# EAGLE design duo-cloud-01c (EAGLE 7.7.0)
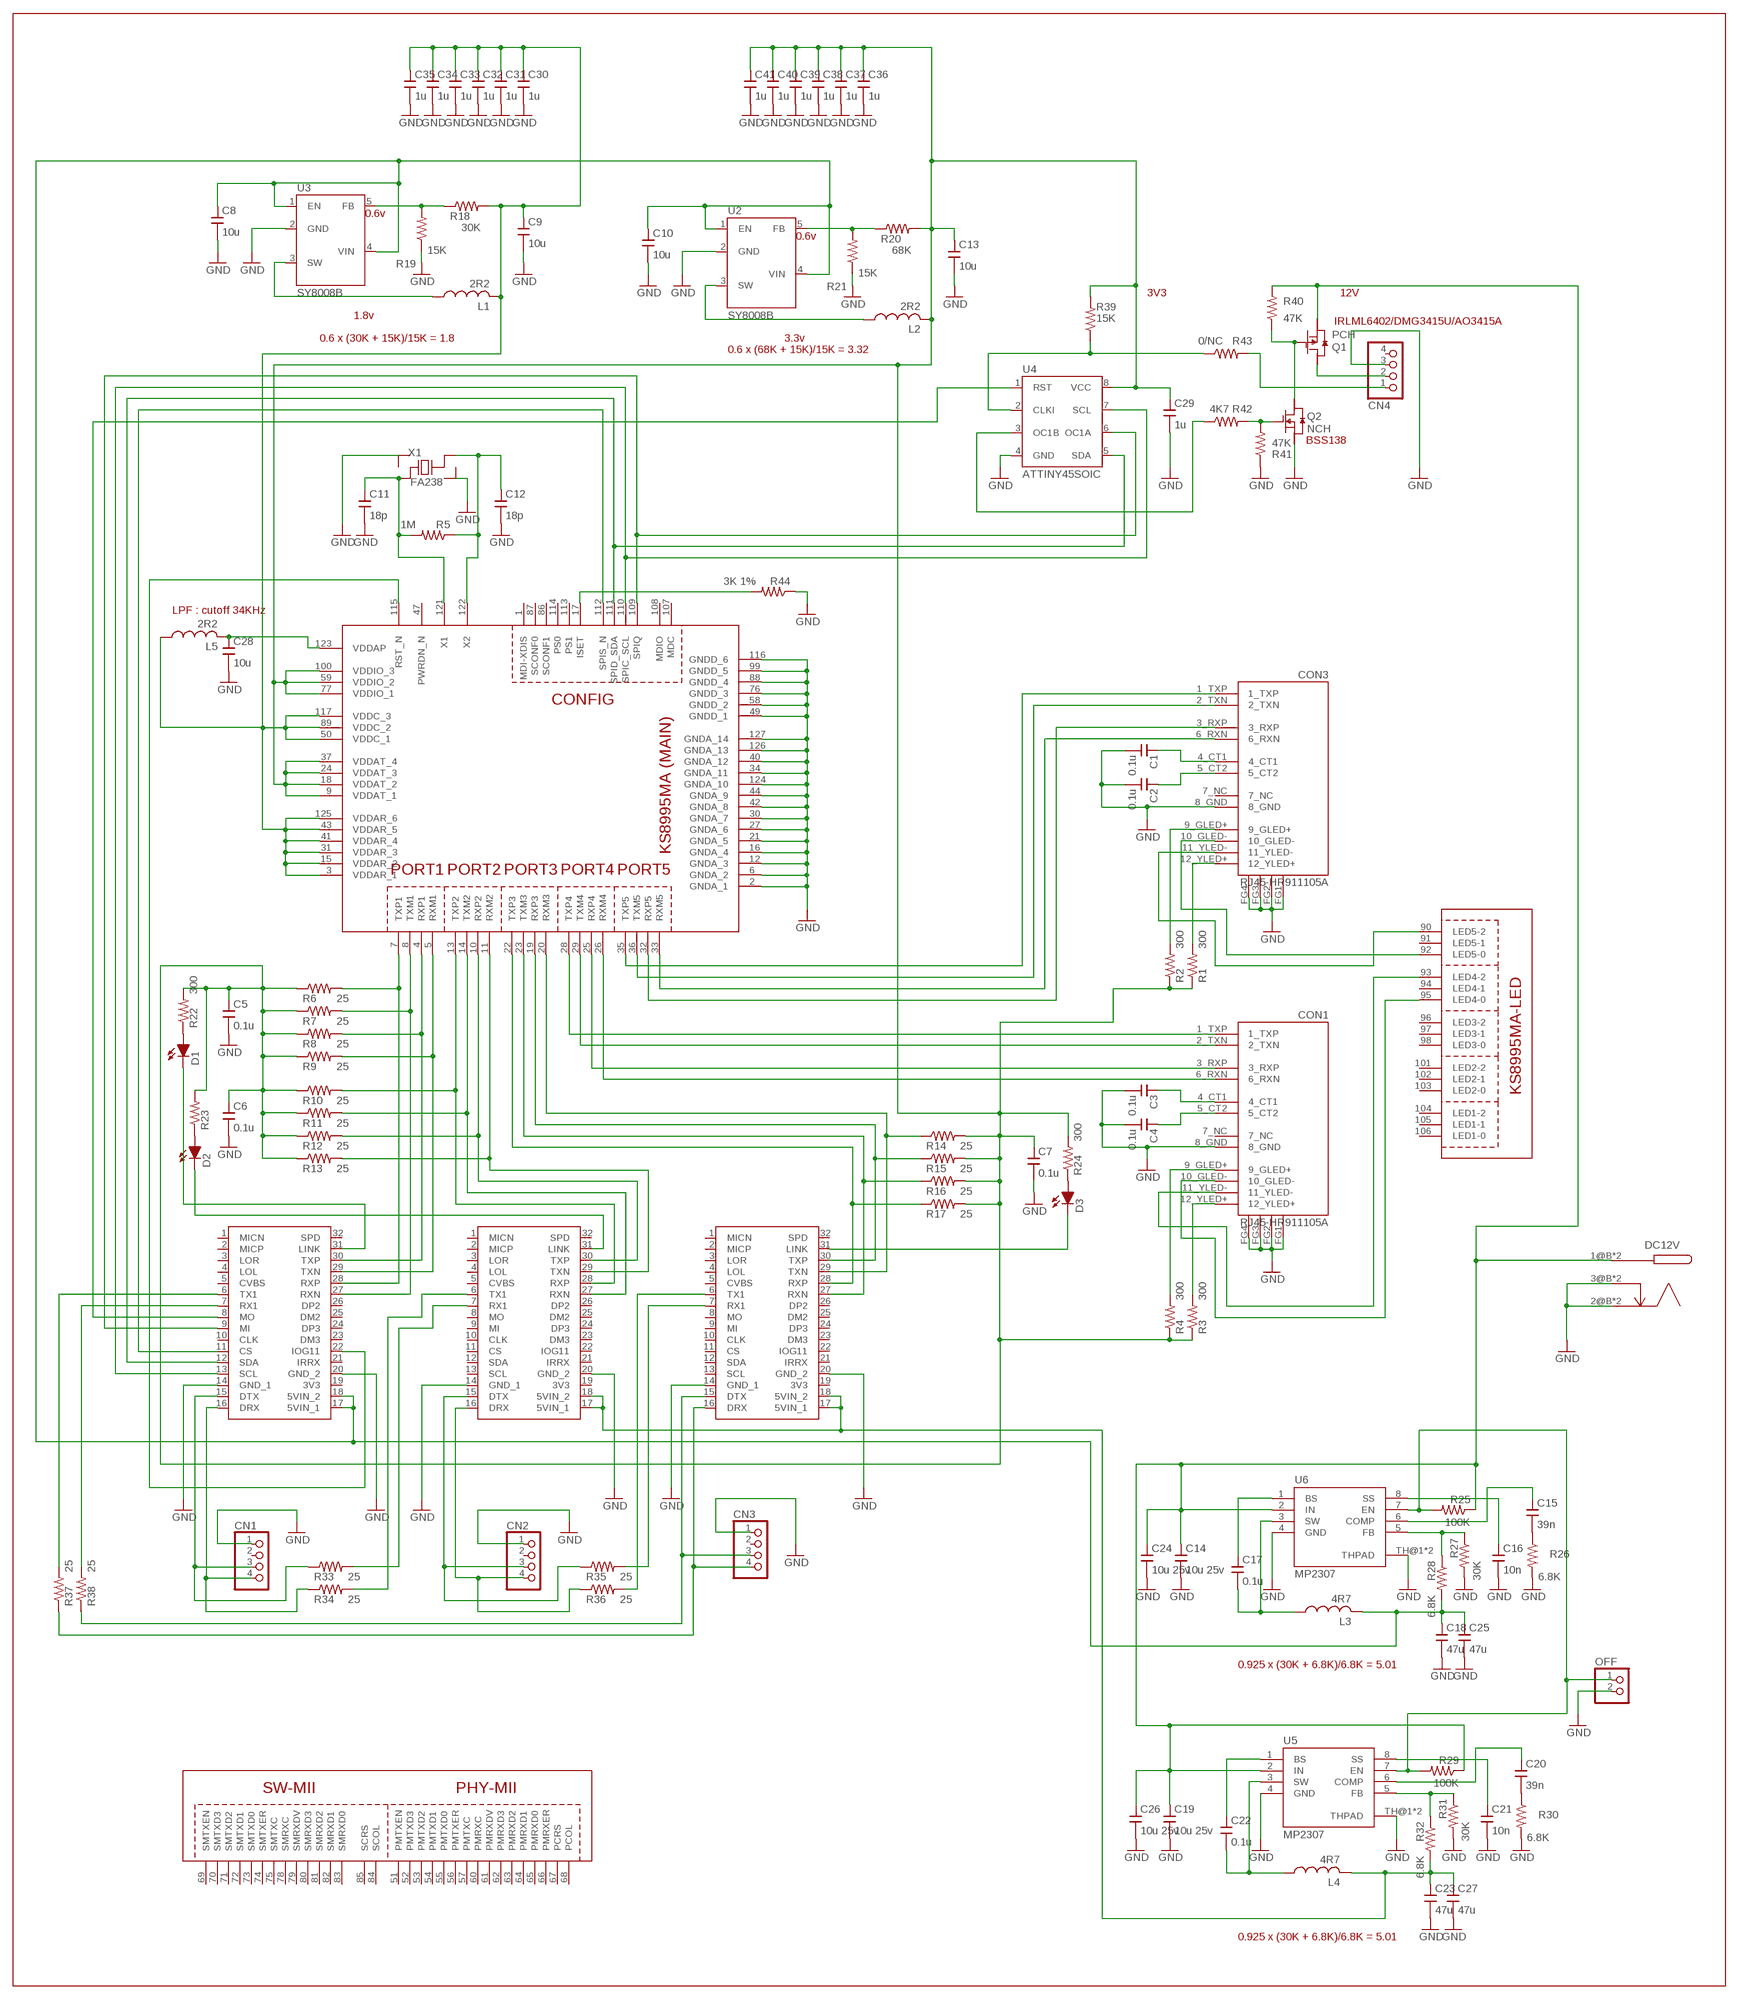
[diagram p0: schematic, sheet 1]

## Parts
C1  0.1u  C/SMDC2012  [C2012]
C2  0.1u  C/SMDC2012  [C2012]
C3  0.1u  C/SMDC2012  [C2012]
C4  0.1u  C/SMDC2012  [C2012]
C5  0.1u  C/SMDC2012  [C2012]
C6  0.1u  C/SMDC2012  [C2012]
C7  0.1u  C/SMDC2012  [C2012]
C8  10u  C/SMDC2012  [C2012]
C9  10u  C/SMDC2012  [C2012]
C10  10u  C/SMDC2012  [C2012]
C11  18p  C/SMDC2012  [C2012]
C12  18p  C/SMDC2012  [C2012]
C13  10u  C/SMDC2012  [C2012]
C14  10u 25v  C/SMDC3216  [C3216]
C15  39n  C/SMDC2012  [C2012]
C16  10n  C/SMDC2012  [C2012]
C17  0.1u  C/SMDC2012  [C2012]
C18  47u  C/SMDC3216  [C3216]
C19  10u 25v  C/SMDC3216  [C3216]
C20  39n  C/SMDC2012  [C2012]
C21  10n  C/SMDC2012  [C2012]
C22  0.1u  C/SMDC2012  [C2012]
C23  47u  C/SMDC3216  [C3216]
C24  10u 25v  C/SMDC3216  [C3216]
C25  47u  C/SMDC3216  [C3216]
C26  10u 25v  C/SMDC3216  [C3216]
C27  47u  C/SMDC3216  [C3216]
C28  10u  C/SMDC2012  [C2012]
C29  1u  C/SMDC2012  [C2012]
C30  1u  C/SMDC2012  [C2012]
C31  1u  C/SMDC2012  [C2012]
C32  1u  C/SMDC2012  [C2012]
C33  1u  C/SMDC2012  [C2012]
C34  1u  C/SMDC2012  [C2012]
C35  1u  C/SMDC2012  [C2012]
C36  1u  C/SMDC2012  [C2012]
C37  1u  C/SMDC2012  [C2012]
C38  1u  C/SMDC2012  [C2012]
C39  1u  C/SMDC2012  [C2012]
C40  1u  C/SMDC2012  [C2012]
C41  1u  C/SMDC2012  [C2012]
CN1  CONN4N  [PINHDR1X4]
CN2  CONN4N  [PINHDR1X4]
CN3  CONN4N  [PINHDR1X4]
CN4  CONN4N  [PINHDR1X4]
CON1  RJ45-HR911105A  [RJ45-HR911105A]
CON3  RJ45-HR911105A  [RJ45-HR911105A]
D1  LED/SMDSMD  [SOD123]
D2  LED/SMDSMD  [SOD123]
D3  LED/SMDSMD  [SOD123]
DC12V  DC-JACK7  [DC-JACK7]
L1  2R2  L/SMDCD54  [CD54]
L2  2R2  L/SMDCD54  [CD54]
L3  4R7  L/SMD  [L10040]
L4  4R7  L/SMD  [L10040]
L5  2R2  L/SMDCD32  [CD32]
M1  NANOPI-DUO  [NANOPI-DUO]
M2  NANOPI-DUO  [NANOPI-DUO]
M3  NANOPI-DUO  [NANOPI-DUO]
OFF  PINHDR2  [PINHDR2]
Q1  PCH  [SOT23]
Q2  NCH  [SOT23]
R1  300  R/SMDR2012  [R2012]
R2  300  R/SMDR2012  [R2012]
R3  300  R/SMDR2012  [R2012]
R4  300  R/SMDR2012  [R2012]
R5  1M  R/SMDR2012  [R2012]
R6  25  R/SMDR2012  [R2012]
R7  25  R/SMDR2012  [R2012]
R8  25  R/SMDR2012  [R2012]
R9  25  R/SMDR2012  [R2012]
R10  25  R/SMDR2012  [R2012]
R11  25  R/SMDR2012  [R2012]
R12  25  R/SMDR2012  [R2012]
R13  25  R/SMDR2012  [R2012]
R14  25  R/SMDR2012  [R2012]
R15  25  R/SMDR2012  [R2012]
R16  25  R/SMDR2012  [R2012]
R17  25  R/SMDR2012  [R2012]
R18  30K  R/SMDR2012  [R2012]
R19  15K  R/SMDR2012  [R2012]
R20  68K  R/SMDR2012  [R2012]
R21  15K  R/SMDR2012  [R2012]
R22  300  R/SMDR2012  [R2012]
R23  300  R/SMDR2012  [R2012]
R24  300  R/SMDR2012  [R2012]
R25  100K  R/SMDR2012  [R2012]
R26  6.8K  R/SMDR2012  [R2012]
R27  30K  R/SMDR2012  [R2012]
R28  6.8K  R/SMDR2012  [R2012]
R29  100K  R/SMDR2012  [R2012]
R30  6.8K  R/SMDR2012  [R2012]
R31  30K  R/SMDR2012  [R2012]
R32  6.8K  R/SMDR2012  [R2012]
R33  25  R/SMDR2012  [R2012]
R34  25  R/SMDR2012  [R2012]
R35  25  R/SMDR2012  [R2012]
R36  25  R/SMDR2012  [R2012]
R37  25  R/SMDR2012  [R2012]
R38  25  R/SMDR2012  [R2012]
R39  15K  R/SMDR2012  [R2012]
R40  47K  R/SMDR2012  [R2012]
R41  47K  R/SMDR2012  [R2012]
R42  4K7  R/SMDR2012  [R2012]
R43  0/NC  R/SMDR2012  [R2012]
R44  3K 1%  R/SMDR2012  [R2012]
U1  KS8995MA+MII  [QFP128]
U2  SY8008B  [SOT235]
U3  SY8008B  [SOT235]
U4  ATTINY45SOIC  [SOIC8]
U5  MP2307  [SOP8PAD]
U6  MP2307  [SOP8PAD]
X1  FA238  [FA238]

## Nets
5VM: C8.1 C10.1 C18.1 C25.1 L3.2 L3.2B M1.17(5VIN_1) M1.18(5VIN_2) R28.2 U2.1(EN) U2.4(VIN) U3.1(EN) U3.4(VIN)
5VS: C23.1 C27.1 L4.2 L4.2B M2.17(5VIN_1) M2.18(5VIN_2) M3.17(5VIN_1) M3.18(5VIN_2) R32.2
CS: M1.11(CS) U1.112(SPIS_N)
GND: C1.2 C2.2 C3.2 C4.2 C5.2 C6.2 C7.2 C8.2 C9.2 C10.2 C11.2 C12.2 C13.2 C14.2 C16.2 C18.2 C19.2 C21.2 C23.2 C24.2 C25.2 C26.2 C27.2 C28.2 C29.2 C30.2 C31.2 C32.2 C33.2 C34.2 C35.2 C36.2 C37.2 C38.2 C39.2 C40.2 C41.2 CN1.1 CN2.1 CN3.1 CN4.3 CON1.8_GND CON1.FG1(GND) CON1.FG2(GND) CON1.FG3(GND) CON1.FG4(GND) CON3.8_GND CON3.FG1(GND) CON3.FG2(GND) CON3.FG3(GND) CON3.FG4(GND) DC12V.2@B(GND) DC12V.2@T(GND) DC12V.3@B(SENSE) DC12V.3@T(SENSE) M1.14(GND_1) M1.20(GND_2) M2.14(GND_1) M2.20(GND_2) M3.14(GND_1) M3.20(GND_2) OFF.2 Q2.2(S) R19.1 R21.1 R26.2 R27.2 R30.2 R31.2 R41.1 R44.1 U1.2(GNDA_1) U1.6(GNDA_2) U1.12(GNDA_3) U1.16(GNDA_4) U1.21(GNDA_5) U1.27(GNDA_6) U1.30(GNDA_7) U1.34(GNDA_11) U1.40(GNDA_12) U1.42(GNDA_8) U1.44(GNDA_9) U1.49(GNDD_1) U1.58(GNDD_2) U1.76(GNDD_3) U1.88(GNDD_4) U1.99(GNDD_5) U1.116(GNDD_6) U1.124(GNDA_10) U1.126(GNDA_13) U1.127(GNDA_14) U2.2(GND) U3.2(GND) U4.4(GND) U5.4(GND) U5.TH@1(THPAD) U5.TH@2(THPAD) U6.4(GND) U6.TH@1(THPAD) U6.TH@2(THPAD) X1.2 X1.4
HUB_1V8: C9.1 C30.1 C31.1 C32.1 C33.1 C34.1 C35.1 L1.2B L1.P$2 L5.1 L5.1B R18.2 U1.3(VDDAR_1) U1.15(VDDAR_2) U1.31(VDDAR_3) U1.41(VDDAR_4) U1.43(VDDAR_5) U1.50(VDDC_1) U1.89(VDDC_2) U1.117(VDDC_3) U1.125(VDDAR_6)
HUB_3V3: C5.1 C6.1 C7.1 C13.1 C29.1 C36.1 C37.1 C38.1 C39.1 C40.1 C41.1 L2.2B L2.P$2 R1.1 R2.1 R3.1 R4.1 R6.1 R7.1 R8.1 R9.1 R10.1 R11.1 R12.1 R13.1 R14.2 R15.2 R16.2 R17.2 R20.2 R22.2 R23.2 R24.2 R39.2 U1.9(VDDAT_1) U1.18(VDDAT_2) U1.24(VDDAT_3) U1.37(VDDAT_4) U1.59(VDDIO_2) U1.77(VDDIO_1) U1.100(VDDIO_3) U4.8(VCC)
HUBRST_N: M1.22(IOG11) U1.115(RST_N)
L1SW: L1.1B L1.P$1 U3.3(SW)
L2SW: L2.1B L2.P$1 U2.3(SW)
MI: M1.9(MI) U1.109(SPIQ) U4.6(OC1A)
N$1: CN4.1 R43.2
N$2: M1.28(RXP) R6.2 U1.7(TXP1)
N$3: M1.27(RXN) R7.2 U1.8(TXM1)
N$4: M1.30(TXP) R8.2 U1.4(RXP1)
N$5: M1.29(TXN) R9.2 U1.5(RXM1)
N$6: M2.28(RXP) R10.2 U1.13(TXP2)
N$7: M2.27(RXN) R11.2 U1.14(TXM2)
N$8: CON3.10_GLED- U1.92(LED5-0)
N$9: M2.30(TXP) R12.2 U1.10(RXP2)
N$10: M2.29(TXN) R13.2 U1.11(RXM2)
N$11: M3.28(RXP) R17.1 U1.22(TXP3)
N$12: M3.27(RXN) R16.1 U1.23(TXM3)
N$13: M3.30(TXP) R15.1 U1.19(RXP3)
N$14: M3.29(TXN) R14.1 U1.20(RXM3)
N$15: CON3.6_RXN U1.33(RXM5)
N$16: CON3.3_RXP U1.32(RXP5)
N$17: CON3.2_TXN U1.36(TXM5)
N$18: CON3.1_TXP U1.35(TXP5)
N$19: C4.1 CON1.5_CT2
N$20: C3.1 CON1.4_CT1
N$21: CON1.9_GLED+ R4.2
N$22: CON1.12_YLED+ R3.2
N$23: OFF.1 R25.2 R29.2 U5.7(EN) U6.7(EN)
N$24: CON1.6_RXN U1.26(RXM4)
N$25: CON1.3_RXP U1.25(RXP4)
N$26: CON1.2_TXN U1.29(TXM4)
N$27: CON1.1_TXP U1.28(TXP4)
N$28: D1.1(A) R22.1
N$29: D2.1(A) R23.1
N$30: D3.1(A) R24.1
N$31: D3.2(C) M3.31(LINK)
N$32: D2.2(C) M2.31(LINK)
N$33: C1.1 CON3.4_CT1
N$34: C2.1 CON3.5_CT2
N$35: D1.2(C) M1.31(LINK)
N$36: CON3.9_GLED+ R2.2
N$37: CON3.12_YLED+ R1.2
N$38: C17.2 L3.1 L3.1B U6.3(SW)
N$39: C17.1 U6.1(BS)
N$40: CON3.11_YLED- U1.90(LED5-2)
N$41: CON1.10_GLED- U1.95(LED4-0)
N$42: CON1.11_YLED- U1.93(LED4-2)
N$43: C28.1 L5.2 L5.2B U1.123(VDDAP)
N$44: CN1.4 M1.16(DRX) R34.1
N$45: C22.2 L4.1 L4.1B U5.3(SW)
N$46: CN1.3 M1.15(DTX) R33.1
N$47: CN3.4 M3.16(DRX) R37.1
N$48: R18.1 R19.2 U3.5(FB)
N$49: C16.1 U6.8(SS)
N$50: C15.2 R26.1
N$51: R20.1 R21.2 U2.5(FB)
N$52: C15.1 U6.6(COMP)
N$53: C11.1 R5.2 U1.121(X1) X1.1
N$54: C12.1 R5.1 U1.122(X2) X1.3
N$55: R27.1 R28.1 U6.5(FB)
N$56: CN2.4 M2.16(DRX) R36.1
N$57: R39.1 R43.1 U4.2(CLKI)
N$58: C21.1 U5.8(SS)
N$59: C20.2 R30.1
N$60: C20.1 U5.6(COMP)
N$61: R31.1 R32.1 U5.5(FB)
N$62: CN2.3 M2.15(DTX) R35.1
N$63: C22.1 U5.1(BS)
N$64: CN3.3 M3.15(DTX) R38.1
N$65: M1.8(MO) U4.1(RST)
N$66: M2.6(TX1) R34.2
N$67: M2.7(RX1) R33.2
N$68: M3.6(TX1) R36.2
N$69: M3.7(RX1) R35.2
N$70: M1.6(TX1) R37.2
N$71: M1.7(RX1) R38.2
N$72: R44.2 U1.17(ISET)
N$73: CN4.2 Q1.3(D)
N$76: Q2.1(G) R41.2 R42.2
N$77: Q1.1(G) Q2.3(D) R40.1
N$78: R42.1 U4.3(OC1B)
SCL: M1.13(SCL) U1.110(SPIC_SCL) U4.7(SCL)
SDA: M1.12(SDA) U1.111(SPID_SDA) U4.5(SDA)
VIN: C14.1 C19.1 C24.1 C26.1 DC12V.1@B(VIN) DC12V.1@T(VIN) Q1.2(S) R25.1 R29.1 R40.2 U5.2(IN) U6.2(IN)
Unconnected: CN1.2 CN2.2 CN3.2 CN4.4 CON1.7_NC CON3.7_NC M1.1(MICN) M1.2(MICP) M1.3(LOR) M1.4(LOL) M1.5(CVBS) M1.10(CLK) M1.19(3V3) M1.21(IRRX) M1.23(DM3) M1.24(DP3) M1.25(DM2) M1.26(DP2) M1.32(SPD) M2.1(MICN) M2.2(MICP) M2.3(LOR) M2.4(LOL) M2.5(CVBS) M2.8(MO) M2.9(MI) M2.10(CLK) M2.11(CS) M2.12(SDA) M2.13(SCL) M2.19(3V3) M2.21(IRRX) M2.22(IOG11) M2.23(DM3) M2.24(DP3) M2.25(DM2) M2.26(DP2) M2.32(SPD) M3.1(MICN) M3.2(MICP) M3.3(LOR) M3.4(LOL) M3.5(CVBS) M3.8(MO) M3.9(MI) M3.10(CLK) M3.11(CS) M3.12(SDA) M3.13(SCL) M3.19(3V3) M3.21(IRRX) M3.22(IOG11) M3.23(DM3) M3.24(DP3) M3.25(DM2) M3.26(DP2) M3.32(SPD) U1.1(MDI-XDIS) U1.47(PWRDN_N) U1.51(PMTXEN) U1.52(PMTXD3) U1.53(PMTXD2) U1.54(PMTXD1) U1.55(PMTXD0) U1.56(PMTXER) U1.57(PMTXC) U1.60(PMRXC) U1.61(PMRXDV) U1.62(PMRXD3) U1.63(PMRXD2) U1.64(PMRXD1) U1.65(PMRXD0) U1.66(PMRXER) U1.67(PCRS) U1.68(PCOL) U1.69(SMTXEN) U1.70(SMTXD3) U1.71(SMTXD2) U1.72(SMTXD1) U1.73(SMTXD0) U1.74(SMTXER) U1.75(SMTXC) U1.78(SMRXC) U1.79(SMRXDV) U1.80(SMRXD3) U1.81(SMRXD2) U1.82(SMRXD1) U1.83(SMRXD0) U1.84(SCOL) U1.85(SCRS) U1.86(SCONF1) U1.87(SCONF0) U1.91(LED5-1) U1.94(LED4-1) U1.96(LED3-2) U1.97(LED3-1) U1.98(LED3-0) U1.101(LED2-2) U1.102(LED2-1) U1.103(LED2-0) U1.104(LED1-2) U1.105(LED1-1) U1.106(LED1-0) U1.107(MDC) U1.108(MDIO) U1.113(PS1) U1.114(PS0)

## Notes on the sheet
- 0.6v
- 0.6v
- 3V3 | 12V
- 1.8v
- IRLML6402/DMG3415U/AO3415A
- 0.6 x (30K + 15K)/15K = 1.8 | 3.3v
- 0.6 x (68K + 15K)/15K = 3.32
- BSS138
- LPF : cutoff 34KHz
- 0.925 x (30K + 6.8K)/6.8K = 5.01
- 0.925 x (30K + 6.8K)/6.8K = 5.01

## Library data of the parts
C1-C41 = SRT162-020:C/SMD
CN1-CN4 = SRT162-020:CONN4: connector 4
CON1 CON3 = SRT162-020:RJ45-HR911105A
D1-D3 = SRT162-020:LED/SMD
DC12V = SRT162-020:DC-JACK
L1-L5 = SRT162-020:L/SMD: VLF4012AT
M1-M3 = SRT162-020:NANOPI-DUO
OFF = SRT162-020:PINHDR2
Q1 = SRT162-020:PCH
Q2 = SRT162-020:NCH
R1-R44 = SRT162-020:R/SMD
U1 = SRT162-020:KS8995MA+MII
U2 U3 = SRT162-020:SY8008B
U4 = SRT162-020:ATTINY45
U5 U6 = SRT162-020:MP2307
X1 = SRT162-020:FA238

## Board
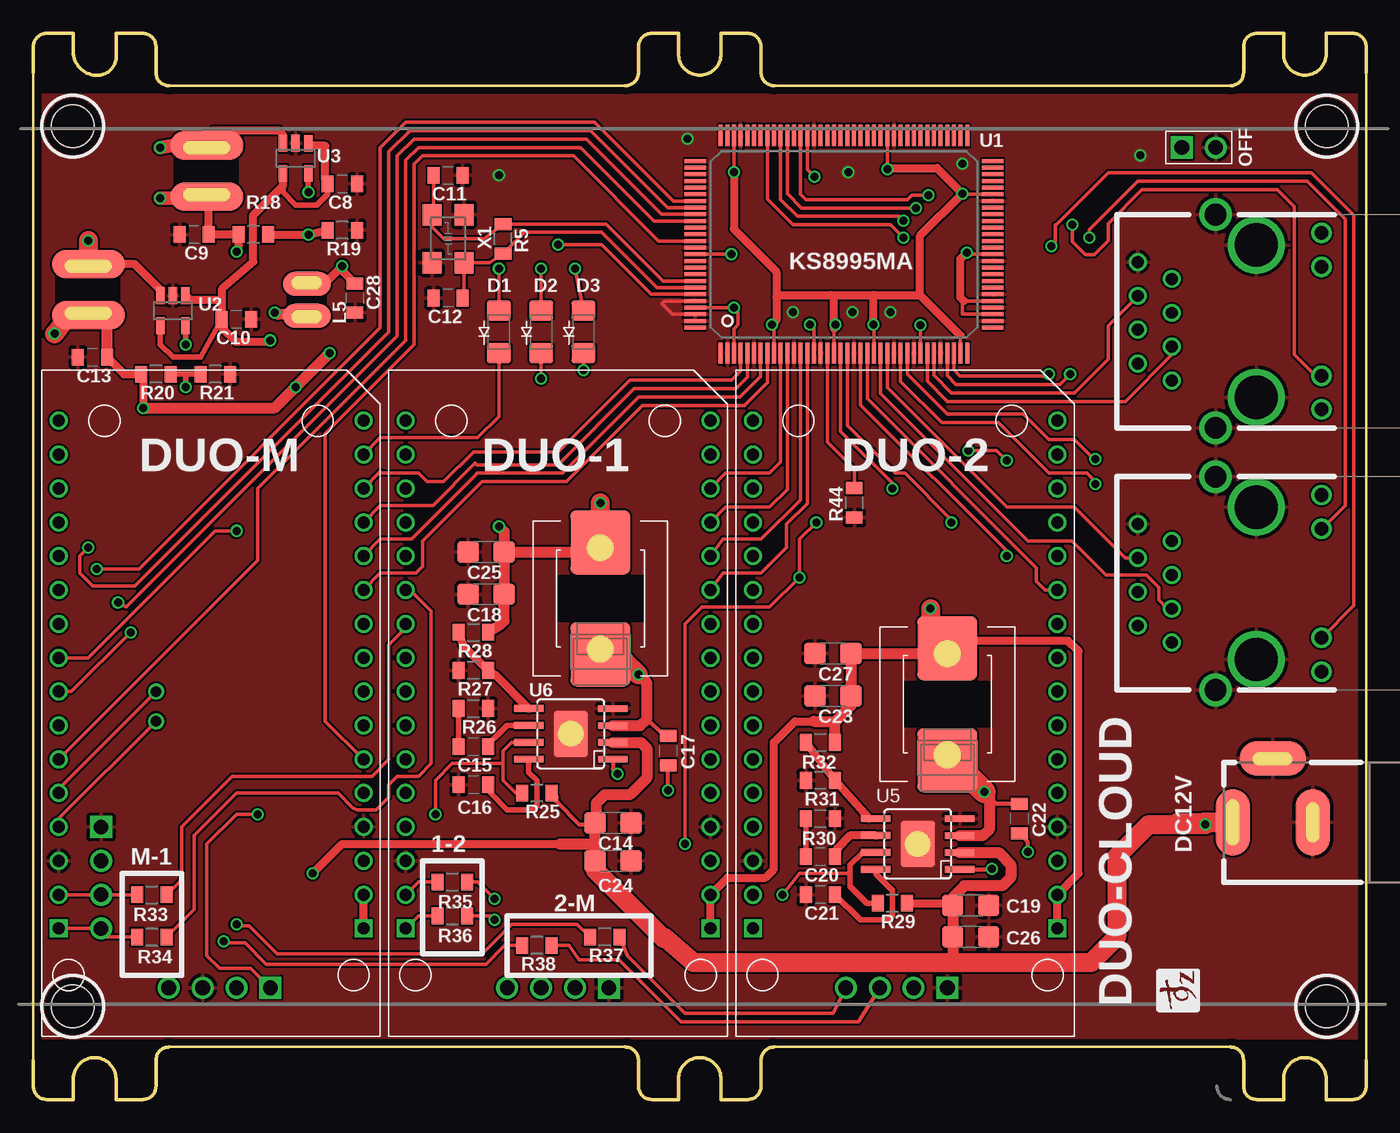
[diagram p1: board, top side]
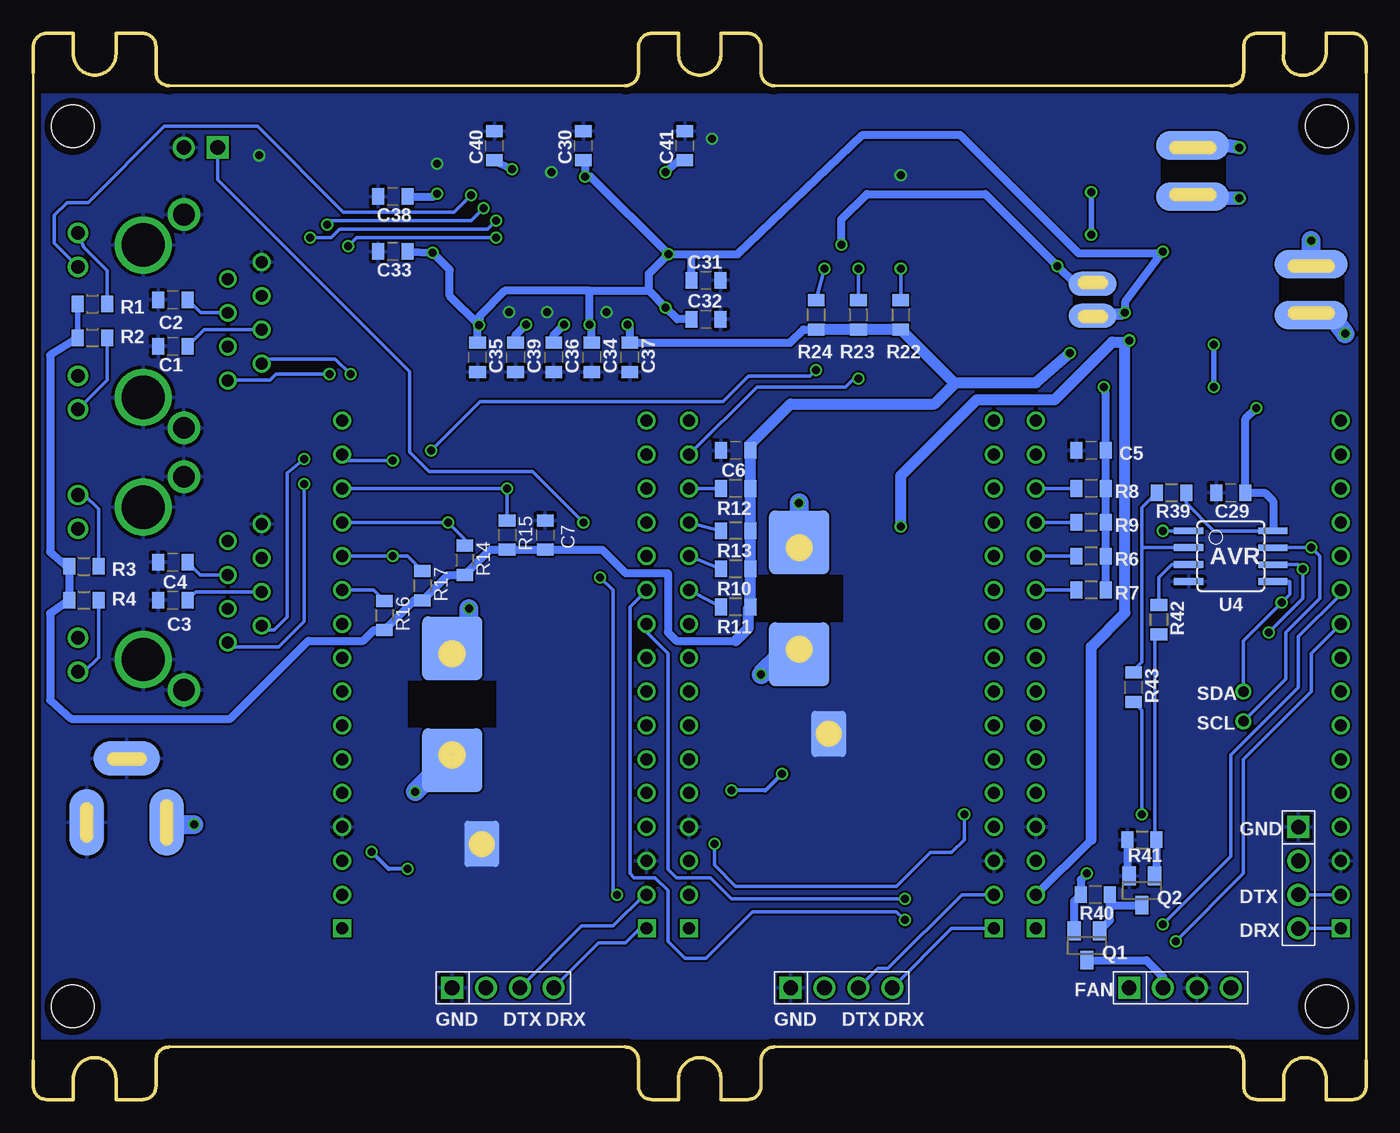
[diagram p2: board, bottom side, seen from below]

Size 100 x 80 mm. Coordinates in mm from the lower left corner, seen from the top.
Outline: 75 segments
Copper layers (1*16): Top 0.035mm / dielectric 1.6mm / Bottom 0.035mm
Design rules "Elecrow_2-layer_PCB_eagle_rule": minimum track width 6mil, minimum drill 12mil, track to track 6mil, track to pad 6mil, pad to pad 6mil, via to via 8mil, smd to smd 0mil, copper to edge 20mil, drill to drill 10mil, minimum pad ring 6mil, minimum via ring 6mil, stop-mask expansion 0mil, vias tented up to drill 100mil, thermal gap 10mil
Holes 3.2 mm at 2.97,73.02 97.05,73.02 2.97,6.98 97.05,6.98
tRestrict: area -4,-1 to 103,4.5; area -3,75.5 to 104,81
bRestrict: area -4,-1 to 103,4.5; area -3,75.5 to 104,81

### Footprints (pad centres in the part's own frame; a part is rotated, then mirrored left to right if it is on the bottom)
C2012 = smd 0.9 x 1.25: 1 -1.1,0; 2 1.1,0
C3216 = smd 1.6 x 1.6: 1 -1.35,0; 2 1.35,0
PINHDR1X4 = drill 1.1 square: 1 -3.81,0 | drill 1.1: 2 -1.27,0; 3 1.27,0; 4 3.81,0
RJ45-HR911105A = drill 0.89 pad 1.144: 1_TXP 4.45,-6.35; 2_TXN 3.18,-8.89; 3_RXP 1.91,-6.35; 4_CT1 0.64,-8.89; 5_CT2 -0.63,-6.35; 6_RXN -1.9,-8.89; 7_NC -3.17,-6.35; 8_GND -4.44,-8.89 | drill 1.02 pad 1.528: 9_GLED+ 6.625,4.9; 10_GLED- 4.085,4.9; 11_YLED- -4.085,4.9; 12_YLED+ -6.625,4.9 | drill 1.63: FG1 8,-3.05; FG2 -8,-3.05 | drill 3.25 pad 3.75: FG3 5.715,0; FG4 -5.715,0
SOD123 = smd 1.5 x 1.8: 1 -1.6,0; 2 1.6,0
DC-JACK7 = smd 2.6 x 5 bottom: 1@B 4,0; 2@B -2,0 | smd 2.6 x 5: 1@T 4,0; 2@T -2,0 | smd 5 x 2.6 bottom: 3@B 1,-4.8 | smd 5 x 2.6: 3@T 1,-4.8
CD54 = smd 5.5 x 2.15 bottom: 1B 0,1.925; 2B 0,-1.925 | smd 5.5 x 2.15: P$1 0,1.925; P$2 0,-1.925
L10040 = smd 4.5 x 4.8: 1 0,4.2; 2 0,-4.2 | smd 4.5 x 4.8 bottom: 1B 0,4.2; 2B 0,-4.2
CD32 = smd 1.8 x 3.6: 1 -1.2,0; 2 1.2,0 | smd 1.8 x 3.6 bottom: 1B -1.2,0; 2B 1.2,0
NANOPI-DUO = drill 0.9: 1 -10.16,10.16; 2 -10.16,7.62; 3 -10.16,5.08; 4 -10.16,2.54; 5 -10.16,0; 6 -10.16,-2.54; 7 -10.16,-5.08; 8 -10.16,-7.62; 9 -10.16,-10.16; 10 -10.16,-12.7; 11 -10.16,-15.24; 12 -10.16,-17.78; 13 -10.16,-20.32; 14 -10.16,-22.86; 15 -10.16,-25.4; 18 12.7,-25.4; 19 12.7,-22.86; 20 12.7,-20.32; 21 12.7,-17.78; 22 12.7,-15.24; 23 12.7,-12.7; 24 12.7,-10.16; 25 12.7,-7.62; 26 12.7,-5.08; 27 12.7,-2.54; 28 12.7,0; 29 12.7,2.54; 30 12.7,5.08; 31 12.7,7.62; 32 12.7,10.16 | drill 0.9 square: 16 -10.16,-27.94; 17 12.7,-27.94
PINHDR2 = drill 1.1 square: 1 -1.27,0 | drill 1.1: 2 1.27,0
SOT23 = smd 1 x 1.4: 1 -0.95,-1.1; 2 0.95,-1.1; 3 0,1.1
R2012 = smd 0.9 x 1.25: 1 -1.1,0; 2 1.1,0
QFP128 = smd 0.3 x 1.6: 1 -9.25,-8.16; 2 -8.75,-8.16; 3 -8.25,-8.16; 4 -7.75,-8.16; 5 -7.25,-8.16; 6 -6.75,-8.16; 7 -6.25,-8.16; 8 -5.75,-8.16; 9 -5.25,-8.16; 10 -4.75,-8.16; 11 -4.25,-8.16; 12 -3.75,-8.16; 13 -3.25,-8.16; 14 -2.75,-8.16; 15 -2.25,-8.16; 16 -1.75,-8.16; 17 -1.25,-8.16; 18 -0.75,-8.16; 19 -0.25,-8.16; 20 0.25,-8.16; 21 0.75,-8.16; 22 1.25,-8.16; 23 1.75,-8.16; 24 2.25,-8.16; 25 2.75,-8.16; 26 3.25,-8.16; 27 3.75,-8.16; 28 4.25,-8.16; 29 4.75,-8.16; 30 5.25,-8.16; 31 5.75,-8.16; 32 6.25,-8.16; 33 6.75,-8.16; 34 7.25,-8.16; 35 7.75,-8.16; 36 8.25,-8.16; 37 8.75,-8.16; 38 9.25,-8.16; 65 9.25,8.16; 66 8.75,8.16; 67 8.25,8.16; 68 7.75,8.16; 69 7.25,8.16; 70 6.75,8.16; 71 6.25,8.16; 72 5.75,8.16; 73 5.25,8.16; 74 4.75,8.16; 75 4.25,8.16; 76 3.75,8.16; 77 3.25,8.16; 78 2.75,8.16; 79 2.25,8.16; 80 1.75,8.16; 81 1.25,8.16; 82 0.75,8.16; 83 0.25,8.16; 84 -0.25,8.16; 85 -0.75,8.16; 86 -1.25,8.16; 87 -1.75,8.16; 88 -2.25,8.16; 89 -2.75,8.16; 90 -3.25,8.16; 91 -3.75,8.16; 92 -4.25,8.16; 93 -4.75,8.16; 94 -5.25,8.16; 95 -5.75,8.16; 96 -6.25,8.16; 97 -6.75,8.16; 98 -7.25,8.16; 99 -7.75,8.16; 100 -8.25,8.16; 101 -8.75,8.16; 102 -9.25,8.16 | smd 1.6 x 0.3: 39 11.16,-6.25; 40 11.16,-5.75; 41 11.16,-5.25; 42 11.16,-4.75; 43 11.16,-4.25; 44 11.16,-3.75; 45 11.16,-3.25; 46 11.16,-2.75; 47 11.16,-2.25; 48 11.16,-1.75; 49 11.16,-1.25; 50 11.16,-0.75; 51 11.16,-0.25; 52 11.16,0.25; 53 11.16,0.75; 54 11.16,1.25; 55 11.16,1.75; 56 11.16,2.25; 57 11.16,2.75; 58 11.16,3.25; 59 11.16,3.75; 60 11.16,4.25; 61 11.16,4.75; 62 11.16,5.25; 63 11.16,5.75; 64 11.16,6.25; 103 -11.16,6.25; 104 -11.16,5.75; 105 -11.16,5.25; 106 -11.16,4.75; 107 -11.16,4.25; 108 -11.16,3.75; 109 -11.16,3.25; 110 -11.16,2.75; 111 -11.16,2.25; 112 -11.16,1.75; 113 -11.16,1.25; 114 -11.16,0.75; 115 -11.16,0.25; 116 -11.16,-0.25; 117 -11.16,-0.75; 118 -11.16,-1.25; 119 -11.16,-1.75; 120 -11.16,-2.25; 121 -11.16,-2.75; 122 -11.16,-3.25; 123 -11.16,-3.75; 124 -11.16,-4.25; 125 -11.16,-4.75; 126 -11.16,-5.25; 127 -11.16,-5.75; 128 -11.16,-6.25
SOT235 = smd 0.635 x 1.27: 1 -0.95,-1.125; 2 0.013,-1.135; 3 0.95,-1.125; 4 0.95,1.125; 5 -0.95,1.125
SOIC8 = smd 0.5 x 2.2: 1 -1.905,-3.154; 2 -0.645,-3.154; 3 0.625,-3.154; 4 1.895,-3.154; 5 1.905,3.154; 6 0.635,3.154; 7 -0.635,3.154; 8 -1.905,3.154
SOP8PAD = smd 0.5 x 2.2: 1 -1.905,-3.154; 2 -0.645,-3.154; 3 0.625,-3.154; 4 1.895,-3.154; 5 1.905,3.154; 6 0.635,3.154; 7 -0.635,3.154; 8 -1.905,3.154 | smd 3.454 x 2.565: TH@1 0,0 | smd 3.454 x 2.565 bottom: TH@2 0,0
FA238 = smd 1.6 x 1.4: 1 -1.8,-1.2; 2 1.8,-1.2; 3 1.8,1.2; 4 -1.8,1.2

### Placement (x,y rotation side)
C1  89.53,56.52 180 bottom
C2  89.53,60.01 180 bottom
C3  89.53,37.47 180 bottom
C4  89.53,40.32 180 bottom
C5  20.64,48.71 180 bottom
C6  47.31,48.71 180 bottom
C7  61.59,42.36 90 bottom
C8  23.18,68.71 0 top
C9  12.06,64.9 180 top
C10  15.24,58.55 0 top
C11  31.11,69.34 0 top
C12  31.11,60.14 180 top
C13  4.45,55.69 180 top
C14  43.5,20.77 0 top
C15  33.02,26.48 180 top
C16  33.02,23.62 180 top
C17  47.62,26.16 90 top
C18  33.97,37.91 180 top
C19  70.33,14.58 0 top
C20  59.05,18.23 180 top
C21  59.05,15.37 180 top
C22  73.98,21.09 90 top
C23  60.01,30.29 180 top
C24  43.5,17.91 0 top
C25  33.97,41.09 180 top
C26  70.33,12.2 0 top
C27  60.01,33.47 180 top
C28  24.13,60.14 270 top
C29  10.16,45.53 180 bottom
C30  58.74,71.57 90 bottom
C31  49.53,61.47 0 bottom
C32  49.53,58.55 0 bottom
C33  73.03,63.63 180 bottom
C34  58.1,55.69 270 bottom
C35  66.67,55.69 270 bottom
C36  60.96,55.69 270 bottom
C37  55.24,55.69 270 bottom
C38  73.03,67.76 180 bottom
C39  63.82,55.69 270 bottom
C40  65.41,71.57 90 bottom
C41  51.12,71.57 90 bottom
CN1  5.08,16.64 270 bottom
CN2  39.37,8.38 0 bottom
CN3  64.77,8.38 0 bottom
CN4  13.97,8.38 0 bottom
CON1  91.76,38.73 270 top
CON3  91.76,58.4 270 top
D1  34.92,57.6 270 top
D2  38.1,57.6 270 top
D3  41.27,57.6 270 top
DC12V  93.98,20.8 180 top
L1  13.02,69.66 0 top
L2  4.13,60.77 0 top
L3  42.55,37.59 180 top
L4  68.58,29.66 180 top
L5  20.51,60.01 90 top
M1  12.06,40.77 0 top
M2  38.1,40.77 0 top
M3  64.14,40.77 0 top
OFF  87.44,71.44 0 top
Q1  20.95,11.56 180 bottom
Q2  16.83,15.69 180 bottom
R1  95.57,59.69 0 bottom
R2  95.57,57.15 0 bottom
R3  96.2,40.01 0 bottom
R4  96.2,37.47 0 bottom
R5  35.24,64.58 90 top
R6  20.64,40.77 180 bottom
R7  20.64,38.23 180 bottom
R8  20.64,45.85 180 bottom
R9  20.64,43.31 180 bottom
R10  47.31,39.82 180 bottom
R11  47.31,36.96 180 bottom
R12  47.31,45.85 180 bottom
R13  47.31,42.67 180 bottom
R14  67.63,40.45 270 bottom
R15  64.45,42.36 270 bottom
R16  73.66,36.33 270 bottom
R17  70.8,38.55 270 bottom
R18  16.51,64.9 180 top
R19  23.18,65.22 180 top
R20  9.21,54.42 180 top
R21  13.65,54.42 180 top
R22  34.92,58.87 270 bottom
R23  38.1,58.87 270 bottom
R24  41.27,58.87 270 bottom
R25  37.78,22.99 180 top
R26  33.02,29.34 0 top
R27  33.02,32.2 180 top
R28  33.02,35.05 0 top
R29  64.45,14.73 180 top
R30  59.05,21.09 0 top
R31  59.05,23.94 180 top
R32  59.05,26.8 0 top
R33  8.89,15.37 0 top
R34  8.89,12.2 0 top
R35  31.43,16.32 0 top
R36  31.43,13.78 0 top
R37  42.86,12.2 180 top
R38  37.78,11.56 180 top
R39  14.61,45.53 0 bottom
R40  20.32,15.37 180 bottom
R41  16.83,19.5 0 bottom
R42  15.56,36.01 270 bottom
R43  17.46,30.93 270 bottom
R44  61.59,44.77 90 top
U1  60.82,64.17 0 top
U2  10.48,59.19 180 top
U3  19.68,70.61 180 top
U4  10.16,40.77 270 bottom
U5  66.36,19.18 90 top
U6  40.32,27.43 90 top
X1  31.11,64.58 270 top

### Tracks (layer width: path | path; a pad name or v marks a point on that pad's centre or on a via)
5VM  (via drill 0.6)
  Top 0.254: 35.01,40.45 35.01,40.69
  Top 0.406: 18.73,68.58 18.73,68.07 19.68,67.12 21.27,67.12 22.08,67.93 C8.1 | 20.81,71.57 U3.1 | 22.23,68.71 21.91,69.03 | U2.4 9.53,56.64 10.48,55.69 12.55,55.69 C10.1 | 35.01,40.69 34.92,40.69
  Top 0.61: 21.91,69.03 21.91,71.57 20.81,71.57 | C8.1 22.23,68.71 | L3.2B 42.94,41.41 | M1.17 M1.18 | L3.2B 42.55,41.27 42.55,40.45 | L3.2B 43.25,41.16 | v17.78,56.96 17.63,56.96 17.5,56.83 15.24,56.83 14.14,57.93 C10.1 14.14,60.01 | U3.4 18.73,68.58 16.51,66.36 16.51,62.85 14.14,60.8 14.14,60.01 | U2.1 11.73,60.01 14.14,60.01 | 35.01,40.69 35.01,40.77 C25.1
  Top 0.813: R28.2 35.01,35.62 35.32,35.94 C18.1 C25.1 | v34.92,42.99 35.32,42.59 C25.1 | C25.1 42.36,41.09 42.55,41.27
  Top 1.422: L3.2B v42.55,44.77
  Top 1.676: 41.52,40.77 L3.2B
  Bottom 0.61: M1.18 20.64,19.5
  Bottom 0.813: v34.92,42.99 34.92,46.8 29.21,52.52 23.36,52.52 19.05,56.83 17.91,56.83 v17.78,56.96 18.1,56.65 18.1,36.51 20.64,33.97 20.64,19.5
  Bottom 1.422: v42.55,44.77 L3.2B 42.55,40.64
5VS  (via drill 0.6)
  Top 0.406: C23.1 61.4,29.62
  Top 0.61: L4.2B 68.78,33.34 69.29,33.15 | 76.52,12.51 M3.17 M3.18 78.42,16.96 78.42,33.66 77.63,34.42 69.17,34.42 L4.2B | L4.2B 68.58,32.52 | M2.17 M2.18 52.07,16.64 54.93,16.64 55.56,17.27 55.56,26.8 57.15,28.39 58.57,28.39
  Top 0.813: C23.1 C27.1 68.19,33.47 L4.2B | 58.57,28.39 60.17,28.39 | 60.17,28.39 61.4,29.62 | R32.2 60.16,28.38 60.17,28.39
  Top 1.422: v67.31,36.83 67.31,34.49 L4.2B
  Bottom 1.422: L4.2B 67.31,33.86 v67.31,36.83
CS
  Top 0.254: M1.11 16.83,40.45 16.83,45.85 27.94,56.96 27.94,70.48 28.89,71.44 41.04,71.44 46.56,65.92 U1.112
GND  (via drill 0.6)
  Top 0.254: U1.124 47.36,59.92 47.17,59.73 47.97,58.92 U1.126
  Bottom 0.254: 17.93,17.25 Q2.2
  Bottom 0.61: R41.1 17.93,17.25
  other vias: 83.05,70.84 49.07,72.11 61.14,69.57 69.71,70.2 61.45,59.09 34.92,69.34 57.01,59.09 64.31,59.09
  pour Bottom: -4.45,86.17 -4.45,-2.82 106.05,-2.82 106.05,86.17
  pour Top: -6.03,87.44 -6.43,-2.2 103.11,-2.2 103.5,88.08 -5.71,88.08
HUB_1V8  (via drill 0.6)
  Top 0.254: U1.117 v52.36,63.42 | U1.125 v52.55,59.42 | v52.55,59.42 52.56,59.41 | U1.3 52.57,57.83 52.88,58.14 52.88,59.09 v52.55,59.42 | U1.15 58.57,57.85 v58.28,58.14 | U1.31 v66.57,58.1 | U1.43 69.83,59.92 69.71,59.92 69.71,58.92 U1.41 | U1.50 70.14,63.42 v70.03,63.53 | U1.89 58.07,69.78 v58.6,69.25
  Top 0.406: v15.24,63.63 15.41,64.09 | 13.16,67.61 13.97,67.44 13.31,67.44 L1.2B
  Top 0.61: 15.41,64.09 R18.2 C9.1 13.16,67.61 | 69.83,59.92 69.55,60.2 69.55,63.06 v70.03,63.53 | L5.1B 18.34,58.81 v18.1,59.05 20.26,59.05 L5.1B
  Top 1.016: v9.53,67.63 12.91,67.63 L1.2B
  Top 1.422: L1.2B 12.38,67.42
  Bottom 0.61: 52.55,63.23 v52.36,63.42 | v66.57,58.1 68.76,60.29 68.76,62.27 v70.03,63.53 C33.1 | 58.28,60.68 64.63,60.68 66.53,58.77 66.53,58.14 v66.57,58.1 | 58.28,60.68 v58.28,58.14 58.1,57.96 C34.1 | v52.36,63.42 50.48,63.42 | 50.48,63.42 47.15,63.42 37.78,72.39 30.48,72.39 21.59,63.5 15.37,63.5 v15.24,63.63 18.1,59.82 v18.1,59.05 | v18.1,59.05 20.26,59.05 L5.1B 18.34,58.81 v18.1,59.05 | C35.1 66.67,58 v66.57,58.1 | v52.36,63.42 58.19,69.25 v58.6,69.25 58.6,70.33 C30.1 | 58.28,60.68 53.81,60.68 | 53.81,60.68 v52.55,59.42 51.68,58.55 C32.1 | 53.81,60.68 53.81,61.97 v52.36,63.42 | C31.1 50.63,63.27 50.48,63.42
  Bottom 1.016: v9.53,67.63 13.02,67.63
  Bottom 1.422: 13.02,67.63 L1.2B
HUB_3V3  (via drill 0.6)
  Top 0.254: U1.59 69.77,67.92 v69.71,67.98 | U1.77 v64.07,69.81 64.31,69.89 | U1.100 52.57,69.89 v52.56,69.57 | U1.9 55.57,57.82 v55.42,58.14 | U1.18 60.07,57.82 v60.19,58.14 | U1.24 63.07,57.82 v63.04,58.14 | U1.37 69.57,57.33
  Top 0.406: 5.54,58.72 5.4,58.87 4.15,58.87 L2.2B
  Top 0.61: 59.87,60.36 55.87,60.36 55.74,60.23 | 59.87,60.36 63.04,60.36 | 63.04,60.36 66.53,60.36 | 66.53,60.36 69.57,57.33 | 60.07,57.82 60.07,60.16 59.87,60.36 | v63.04,58.14 63.04,60.36 | 64.31,69.89 67.81,69.89 v69.71,67.98 66.53,64.81 66.53,60.36 | v52.56,69.57 52.56,65.31 55.74,62.13 55.74,60.23 | 55.74,60.23 55.74,58.45 v55.42,58.14 | C13.1 6.82,54.42 R20.2 8.26,54.27 v8.26,51.88
  Top 0.813: C13.1 5.54,58.72 | v22.23,56.01 v19.68,53.47 18.1,51.88 v8.26,51.88
  Top 1.422: L2.2B 2.65,58.85 v1.59,57.47
  Bottom 0.254: 46.35,37.91 46.52,38.06 R11.1 | v64.07,69.81 64.24,69.81 | 6.99,42.7 U4.8 11.43,42.67 13.51,44.75 R39.2
  Bottom 0.406: R1.1 R2.1 | R3.1 97.47,40.01 97.3,39.84
  Bottom 0.61: R7.1 R6.1 R9.1 R8.1 C5.1 19.54,52.98 v19.68,53.47 | 6.99,42.7 6.99,44.9 7.62,45.53 C29.1 9.06,51.08 v8.26,51.88 | 30.95,53.79 30.8,53.79 | C6.1 46.21,49.17 | 46.35,36.96 46.35,37.91 | R2.1 98.74,55.84 98.74,41.09 97.47,40.01 | 97.3,39.84 R4.1 98.74,36.47 98.74,29.98 97.16,28.57 85.22,28.57 79.38,34.42 75.25,34.42 74.44,35.23 R16.2 71.44,37.45 R17.2 68.9,39.35 R14.2 65.72,41.26 R15.2 C7.1 57.32,41.26 55.56,39.5 52.39,39.5 52.39,35.05 51.75,34.42 47.31,34.42 | 46.35,36.81 R11.1 | 40.96,57.77 R24.2 41.29,57.78 42.23,57.78 43.22,56.79 C37.1 55.24,57.96 v55.42,58.14 | C39.1 63.82,57.36 v63.04,58.14 | C36.1 60.96,57.36 v60.19,58.14 | C38.1 69.93,67.76 v69.71,67.98 | C41.1 51.49,70.52 v52.56,69.57 | C40.1 65.38,70.44 v64.07,69.81
  Bottom 0.813: 40.96,57.77 R23.2 R22.2 30.95,53.79 | R11.1 R10.1 R13.1 R12.1 C6.1 | v22.23,56.01 24.77,53.79 30.8,53.79 32.38,52.2 43.18,52.2 46.21,49.17 | 47.31,34.42 46.35,35.37 46.35,36.81
  Bottom 1.422: v1.59,57.47 2.65,58.85 L2.2B
HUBRST_N
  Top 0.254: M1.22 21.91,28.39 21.91,49.98 28.57,56.65 28.57,70.17 29.21,70.8 40.53,70.8 46.92,64.42 U1.115
L1SW  (via drill 0.6)
  Top 0.406: 18.73,72.2 | 13.04,72.2 L1.1B
  Top 0.61: U3.3 18.73,72.2 18.73,72.39 18.41,72.71 13.5,72.71 L1.1B
  Top 1.016: v9.53,71.44 13.02,72.07
  Top 1.422: 13.02,72.07 L1.1B
  Bottom 1.016: v9.53,71.44 12.87,72.07 L1.1B
L2SW  (via drill 0.6)
  Top 0.406: 4.15,62.68 L2.1B
  Top 0.61: U2.3 9.53,60.77 7.62,62.68 4.15,62.68
  Top 1.422: v4.13,64.45 L2.1B
  Bottom 1.422: L2.1B v4.13,64.45
MI  (via drill 0.6)
  Top 0.254: v4.76,39.82 7.94,39.82 26.04,57.91 26.04,71.44 27.94,73.34 42.12,73.34 48.05,67.42 U1.109 | v7.3,35.05 2.86,30.61 M1.9
  Bottom 0.254: U4.6 5.08,40.13 v4.76,39.82 4.76,37.59 v7.3,35.05
N$1  (via drill 0.6)
  Top 0.254: v16.83,21.4 15.24,21.4 13.02,19.18 13.02,10.79 13.97,9.84 16.32,9.84 CN4.1
  Bottom 0.254: R43.2 16.83,29.19 v16.83,21.4
N$2
  Top 0.254: M1.28 26.04,42.04 28.39,42.04 33.15,46.8 33.28,46.99 39.69,46.99 45.4,52.7 53.02,52.7 54.57,54.25 U1.7
  Bottom 0.254: R6.2 M1.28
N$3
  Top 0.254: M1.27 26.04,39.5 28.7,39.5 29.21,40.01 29.21,41.91 33.66,46.35 40.01,46.35 45.72,52.07 53.34,52.07 55.07,53.8 U1.8
  Bottom 0.254: R7.2 M1.27
N$4
  Top 0.254: M1.30 26.04,47.12 26.16,46.99 28.89,46.99 29.53,46.35 30.8,46.35 33.02,48.58 39.37,48.58 44.77,53.98 52.39,53.98 53.07,54.66 U1.4
  Bottom 0.254: R8.2 M1.30
N$5
  Top 0.254: M1.29 26.04,44.58 29.98,44.58 33.15,47.76 33.28,47.62 39.37,47.62 45.09,53.34 52.7,53.34 53.57,54.2 U1.5
  Bottom 0.254: R9.2 M1.29
N$6
  Top 0.254: M2.28 51.75,42.04 54.61,42.04 57.57,45 U1.13
  Bottom 0.254: R10.2 M2.28
N$7
  Top 0.254: M2.27 51.75,39.5 54.61,39.5 56.52,41.41 56.52,43.18 58.07,44.73 U1.14
  Bottom 0.254: R11.2 M2.27
N$8  (via drill 0.6)
  Top 0.254: CON3.10_GLED- 96.18,54.31 94.61,55.88 94.61,66.99 93.34,68.26 83.19,68.26 80.64,65.72 80.64,64.45 79.6,63.41 78.92,63.41 77.97,64.36 v77.97,65.63 | U1.92 56.57,67.97 57.65,66.9 v66.22,66.9
  Bottom 0.254: v66.22,66.9 67.17,65.94 77.65,65.94 v77.97,65.63
N$9
  Top 0.254: U1.10 56.07,47.81 55.24,46.99 51.94,46.99 M2.30
  Bottom 0.254: R12.2 M2.30
N$10
  Top 0.254: U1.11 56.57,45.77 55.24,44.45 51.94,44.45 M2.29
  Bottom 0.254: R13.2 M2.29
N$11  (via drill 0.6)
  Top 0.254: U1.22 62.07,52.12 73.03,41.17 v73.03,40.77
  Bottom 0.254: M3.28 v73.03,40.77 71.92,40.77 R17.1
N$12
  Top 0.254: U1.23 62.57,52.58 75.25,39.9 75.25,38.87 75.88,38.23 M3.27
  Bottom 0.254: R16.1 74.47,38.23 M3.27
N$13  (via drill 0.6)
  Top 0.254: U1.19 60.57,50.13 64.45,46.25 v64.45,45.85
  Bottom 0.254: M3.30 v64.45,45.85 R15.1
N$14  (via drill 0.6)
  Top 0.254: U1.20 61.07,50.59 64.67,46.99 65.41,46.99 68.9,43.5 v68.9,43.31
  Bottom 0.254: M3.29 v68.9,43.31 67.63,42.04 R14.1
N$15
  Top 0.254: CON3.6_RXN 80.64,58.08 80.64,55.56 78.11,53.02 68.9,53.02 67.57,54.35 U1.33
N$16
  Top 0.254: CON3.3_RXP 85.41,55.88 81.92,52.39 68.58,52.39 67.07,53.9 U1.32
N$17  (via drill 0.6)
  Top 0.254: U1.36 69.07,54.76 69.53,54.29 76.07,54.29 v76.2,54.42
  Bottom 0.254: 82.58,54.93 CON3.2_TXN 82.58,55.22 82.23,55.56 77.34,55.56 v76.2,54.42
N$18  (via drill 0.6)
  Top 0.254: v77.79,54.42 77.02,53.66 69.22,53.66 68.57,54.3 U1.35
  Bottom 0.254: v77.79,54.42 81.78,54.42 82.23,53.98 85.38,53.98 CON3.1_TXP
N$19
  Bottom 0.254: CON1.5_CT2 87.48,39.37 C4.1
N$20
  Bottom 0.254: CON1.4_CT1 87.81,38.09 C3.1
N$21
  Bottom 0.254: R4.2 95.1,33.17 96.2,32.07 96.61,32.07 CON1.9_GLED+
N$22
  Bottom 0.254: R3.2 95.1,44.3 96.2,45.4 96.61,45.4 CON1.12_YLED+
N$23  (via drill 0.6)
  Top 0.254: 61.28,16.96 57.47,16.96 v56.2,15.37 | v58.74,43.31 57.47,42.04 v57.47,39.18 55.24,36.96 50.16,36.96 48.9,35.69 v48.9,19.18 | U6.7 35.88,26.8 35.24,26.16 35.24,25.21 | R25.2 36.2,22.99 35.24,23.94 35.24,25.21 | 35.24,25.21 31.43,25.21 30.16,23.94 v30.16,21.4
  Top 0.406: R29.2 62.55,14.73 61.28,16 61.28,16.96 61.28,17.59 62.23,18.55 U5.7
  Bottom 0.254: v56.2,15.37 56.52,15.37 56.52,38.23 v57.47,39.18 | v30.16,21.4 30.16,19.5 31.11,18.55 32.7,18.55 35.24,16 47.31,16 48.9,17.59 v48.9,19.18 | v58.74,43.31 62.55,47.12 70.3,47.12 71.75,48.58 71.75,54.61 86.17,69.03 OFF.1
N$24
  Top 0.254: U1.26 64.07,53.41 73.03,44.45 78.11,44.45 81.92,40.63 CON1.6_RXN
N$25
  Top 0.254: U1.25 63.57,52.95 74.61,41.91 77.92,41.91 80.46,39.37 83.5,39.37 84.45,38.42 84.45,37.47 85.09,36.83 CON1.3_RXP
N$26  (via drill 0.6)
  Top 0.254: v79.69,48.07 79.56,48.07 78.11,49.53 76.2,49.53 74.3,51.44 68.58,51.44 65.57,54.45 U1.29
  Bottom 0.254: CON1.2_TXN 82.56,35.24 81.92,35.24 80.96,36.2 80.96,46.99 v79.69,48.07
N$27  (via drill 0.6)
  Top 0.254: U1.28 65.07,53.89 68.16,50.8 72.39,50.8 76.2,46.99 79.06,46.99 79.69,46.35 v79.69,46.17
  Bottom 0.254: CON1.1_TXP 85.09,33.97 81.6,33.97 79.69,35.88 v79.69,46.17
N$28  (via drill 0.6)
  Top 0.254: v34.92,62.36 D1.1
  Bottom 0.254: R22.1 v34.92,62.36
N$29  (via drill 0.6)
  Top 0.254: D2.1 v38.1,62.36
  Bottom 0.254: v38.1,62.36 R23.1
N$30  (via drill 0.6)
  Top 0.254: D3.1 v40.64,62.36
  Bottom 0.254: v40.64,62.36 R24.1
N$31  (via drill 0.6)
  Top 0.254: v41.27,54.74 D3.2 | v73.03,47.94 72.26,48.71 v70.17,48.71
  Bottom 0.254: v41.27,54.74 41.72,54.29 46.35,54.29 48.26,52.39 66.49,52.39 v70.17,48.71 | M3.31 76.39,47.94 v73.03,47.94
N$32  (via drill 0.6)
  Top 0.254: v38.1,54.1 D2.2
  Bottom 0.254: M2.31 45.72,53.47 39.05,53.47 38.42,54.1 v38.1,54.1
N$33
  Bottom 0.254: CON3.4_CT1 87.19,57.76 C1.1
N$34
  Bottom 0.254: CON3.5_CT2 87.46,59.03 C2.1
N$35
  Top 0.254: M1.31 26.04,49.66 33.34,49.66 34.92,51.25 D1.2
N$36
  Bottom 0.254: R2.2 94.47,53.97 CON3.9_GLED+
N$37
  Bottom 0.254: R1.2 94.47,62.21 96.2,63.95 96.59,64.9 CON3.12_YLED+
N$38  (via drill 0.6)
  Top 0.305: C17.2 47.35,27.27 46.04,28.57
  Top 0.406: L3.1B 44.41,32.87
  Top 0.813: U6.3 45.52,28.06 46.04,28.57 46.04,31.25 v45.4,31.88
  Top 1.016: 45.59,31.88 v45.4,31.88
  Top 1.422: 44.41,32.87 v45.4,31.88 | 43.89,33.4 L3.1B
  Bottom 1.422: L3.1B 43.89,33.4 v45.4,31.88
N$39  (via drill 0.6)
  Top 0.305: U6.1 43.48,24.79 v43.81,24.45 | v47.62,23.18 C17.1
  Bottom 0.305: v43.81,24.45 45.09,23.18 v47.62,23.18
N$40  (via drill 0.6)
  Top 0.254: U1.90 57.57,67.92 57.96,67.53 65.58,67.53 65.9,67.85 v67.17,67.85
  Bottom 0.254: CON3.11_YLED- 98.42,64.25 98.42,66.36 97.47,67.31 95.89,67.31 90.17,73.03 83.19,73.03 76.74,66.58 68.44,66.58 v67.17,67.85
N$41  (via drill 0.6)
  Top 0.254: U1.95 55.07,67.57 57.01,65.63 64.31,65.63 v65.27,64.67 | CON1.10_GLED- 99.06,37.05 99.06,66.36 95.89,69.53 80.64,69.53 76.74,65.63 76.69,65.63 76.69,64.36 v76.38,64.04
  Bottom 0.254: v65.27,64.67 75.74,64.67 v76.38,64.04
N$42  (via drill 0.6)
  Top 0.254: U1.93 56.07,67.52 57.33,66.26 64.95,66.26 v65.27,65.94 | CON1.11_YLED- 98.42,44.59 98.42,66.04 95.57,68.9 82.87,68.9 79.23,65.27 v79.23,64.67
  Bottom 0.254: v65.27,65.94 65.9,65.31 77.01,65.31 77.65,64.67 v79.23,64.67
N$43  (via drill 0.6)
  Top 0.254: 21.91,61.34 L5.2 | U1.123 46.34,60.42 42.63,64.14 v39.37,64.14
  Top 0.61: C28.1 23.18,62.19 v23.18,62.55 | L5.2 21.84,61.21 v23.18,62.55 | 21.91,61.34 21.97,61.34 v23.18,62.55
  Bottom 0.61: v39.37,64.14 39.37,66.04 37.47,67.94 28.57,67.94 v23.18,62.55 21.84,61.21 L5.2
N$44
  Top 0.254: R34.1 5.4,12.2 5.4,12.83 M1.16
  Bottom 0.254: M1.16 CN1.4
N$45  (via drill 0.6)
  Top 0.305: C22.2 72.24,22.18 v71.34,23.08
  Top 0.406: L4.1B 69.81,24.62
  Top 0.813: U5.3 71.24,19.8 71.75,20.32 71.75,22.67 v71.34,23.08
  Top 1.422: v71.34,23.08 68.97,25.46 L4.1B
  Top 1.676: 69.81,24.62 v71.34,23.08
  Bottom 1.422: L4.1B 68.97,25.46 v71.34,23.08
N$46
  Top 0.254: R33.1 M1.15
  Bottom 0.254: M1.15 CN1.3
N$47
  Top 0.254: CN3.4 60.01,6.48 48.9,6.48 44.6,10.78 R37.1
  Bottom 0.254: CN3.4 57.6,11.75 55.56,11.75 54.48,12.83 M3.16
N$48  (via drill 0.6)
  Top 0.406: U3.5 20.64,68.39 v20.64,68.08
  Top 0.61: R18.1 v20.64,64.9 20.81,64.9 R19.2
  Bottom 0.406: v20.64,68.08 v20.64,64.9
N$49
  Top 0.406: U6.8 37.17,24.56 37.78,23.94 37.78,22.04 37.47,21.72 35.56,21.72 34.29,22.99 34.29,23.45 C16.1
N$50
  Top 0.406: R26.1 C15.2
N$51  (via drill 0.6)
  Top 0.406: U2.5 11.43,56.96 v11.43,56.65 | v11.43,53.47 11.43,54.42 | 11.43,54.42 R21.2 | R20.1 11.43,54.42
  Bottom 0.406: v11.43,56.65 v11.43,53.47
N$52
  Top 0.406: U6.6 35.56,28.07 34.61,27.12 33.97,26.63 C15.1
N$53
  Top 0.254: R5.2 33.83,64.58 30.8,64.58 29.91,65.47 X1.1 30.02,66.48 C11.1 | U1.121 47.25,61.42 42.98,65.68 R5.2 | 35.28,65.72 R5.2
N$54
  Top 0.254: C12.1 32.31,60.24 X1.3 34.23,62.78 R5.1 36.85,65.09 42.63,65.09 46.8,60.92 U1.122
N$55
  Top 0.61: U6.5 34.63,31.88 R27.1 32.24,34.08 R28.1
N$56
  Top 0.254: R36.1 28.89,13.78 M2.16
  Bottom 0.254: M2.16 31.11,12.83 CN2.4
N$57
  Bottom 0.254: R39.1 16.83,44.41 16.83,41.41 | 16.83,41.41 16.83,32.83 17.46,32.2 R43.1 | U4.2 16.82,41.41 16.83,41.41
N$58
  Top 0.406: U5.8 63.2,16.94 64.45,15.69 64.45,13.78 64.14,13.46 62.06,13.46 C21.1
N$59
  Top 0.406: R30.1 C20.2
N$60
  Top 0.406: 60.33,18.86 60.33,18.38
  Top 0.61: U5.6 61.28,19.82 60.33,18.86 | 60.33,18.38 C20.1
N$61
  Top 0.406: 62.7,21.09 U5.5 | 60.16,23.96 R31.1
  Top 0.61: R31.1 62.7,21.09 | R32.1 60.16,23.96
N$62
  Top 0.254: M2.15 28.89,16.32 R35.1
  Bottom 0.254: M2.15 30.35,15.37 35.88,9.84 36.64,9.84 CN2.3
N$63  (via drill 0.6)
  Top 0.305: U5.1 71.89,17.27 v71.91,17.3 | v74.61,18.57 74.61,19.35 C22.1
  Bottom 0.305: v71.91,17.3 73.34,17.3 v74.61,18.57
N$64
  Top 0.254: CN3.3 61.91,5.84 48.58,5.84 43.95,10.48 40.96,10.48 40.19,11.56 R38.1
  Bottom 0.254: CN3.3 58.87,13.02 56.52,13.02 54.16,15.37 M3.15
N$65  (via drill 0.6)
  Top 0.254: v15.24,42.67 13.65,42.67 4.13,33.15 M1.8
  Bottom 0.254: U4.1 v15.24,42.67
N$66
  Top 0.254: M2.6 28.26,38.23 29.84,36.64 29.84,25.21 28.89,24.26 27.3,24.26 26.67,23.62 26.67,22.67 25.72,21.72 24.28,21.72 23.96,21.89 22.86,22.99 15.24,22.99 12.06,19.82 12.06,14.27 R34.2
N$67
  Top 0.254: M2.7 27.94,35.37 26.67,34.1 26.67,25.53 25.4,24.26 14.92,24.26 11.11,20.45 11.11,16.49 R33.2
N$68  (via drill 0.6)
  Top 0.254: R36.2 34.29,13.78 v34.61,13.46
  Bottom 0.254: M3.6 55.24,36.96 55.24,16.96 54.93,16.64 53.34,16.64 52.39,15.69 52.39,11.88 51.12,10.61 49.53,10.61 46.04,14.1 35.24,14.1 v34.61,13.46
N$69  (via drill 0.6)
  Top 0.254: R35.2 33.34,16.32 v34.61,15.05
  Bottom 0.254: M3.7 53.98,35.05 52.39,33.47 52.39,17.27 51.75,16.64 49.21,16.64 47.62,15.05 v34.61,15.05
N$70  (via drill 0.6)
  Top 0.254: R37.2 40.81,13.15 35.88,13.15 33.66,10.93 18.29,10.93 16.19,13.02 15.37,13.02 v15.24,13.15
  Bottom 0.254: M1.6 1.91,37.91 5.08,34.74 5.08,30.93 10.16,25.85 10.16,18.23 v15.24,13.15
N$71  (via drill 0.6)
  Top 0.254: R38.2 35.37,11.56 33.97,10.16 17.46,10.16 15.88,11.75 14.42,11.75 v14.29,11.88
  Bottom 0.254: M1.7 4.13,33.47 4.13,30.61 9.21,25.53 9.21,16.96 v14.29,11.88
N$72
  Top 0.254: U1.17 59.57,49.33 61.59,47.31 R44.2
N$73
  Bottom 0.61: Q1.3 16.49,10.46 15.24,9.21 CN4.2
N$76
  Bottom 0.254: R42.2 15.88,34.59 15.88,19.64 R41.2 | 15.73,17.25 Q2.1
  Bottom 0.61: R41.2 15.73,17.25
N$77
  Bottom 0.254: 16.98,15.05 Q2.3
  Bottom 0.61: Q1.1 19.22,13.45 R40.1 19.07,14.59 Q2.3
N$78
  Bottom 0.254: U4.3 14.6,40.15 15.56,39.18 R42.1
SCL  (via drill 0.6, 0.8)
  Top 0.254: v4.13,41.41 3.49,40.77 3.49,39.5 4.45,38.55 7.62,38.55 26.67,57.6 26.67,71.12 28.26,72.71 41.8,72.71 47.59,66.92 U1.110 | v9.21,28.39 1.91,21.09 M1.13
  Bottom 0.254: U4.7 v4.13,41.41 3.49,40.77 3.49,37.59 6.03,35.05 6.03,31.56 v9.21,28.39
SDA  (via drill 0.6, 0.8)
  Top 0.254: v6.35,37.28 6.99,36.96 27.3,57.28 27.3,70.8 28.57,72.07 41.49,72.07 47.14,66.42 U1.111 | v9.21,30.61 1.91,23.31 M1.12
  Bottom 0.254: U4.5 5.71,38.87 5.71,37.91 v6.35,37.28 9.21,34.42 v9.21,30.61
VIN  (via drill 0.6)
  Top 0.305: 39.2,22.67 39.2,22.39 40.96,20.64 42.15,20.64 C14.1
  Top 0.406: R25.1 39.2,22.67
  Top 0.61: R29.1 68.82,14.73 C19.1 | v20.95,16.96 23.18,19.18 39.5,19.18 | 42.02,20.64 C14.1
  Top 0.813: U6.2 45.6,26.79 46.04,26.35 46.04,24.13 44.77,22.86 42.86,22.86 42.23,22.23 42.23,20.85 C14.1 42.15,19.18 | U5.2 72.43,18.54 73.34,17.62 73.34,16.67 72.71,16.03 69.85,16.03 69.06,15.24 69.06,14.66 C19.1 | C19.1 C26.1 | C19.1 68.98,10.05 69.06,10.29 | 39.5,19.18 42.15,19.18 | 42.15,19.18 C24.1
  Top 1.422: 87.79,20.8 DC12V.1@B 85.89,20.8 v87.95,20.64 83.69,20.64 81.28,18.23 81.28,12.2 79.38,10.29 69.06,10.29 49.53,10.29 47.31,12.2 47.31,12.06 42.15,17.23 C24.1
  Bottom 0.61: Q1.2 21.91,14.88 R40.2 21.42,16.49 v20.95,16.96
  Bottom 1.422: DC12V.1@B 89.82,20.64 v87.95,20.64

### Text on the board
tPlace: KS8995MA | DUO-M | DUO-1 | DUO-2 | 1-2 | M-1 | 2-M | DUO-CLOUD
bPlace: AVR | SDA | SCL | GND | DTX | DRX | FAN | DRX | DTX | GND | DRX | DTX | GND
